FUNCTION "Analog I/O convert" : VOID
TITLE =ANALOGUE I/O MANAGEMENT
AUTHOR : Diego_M
VERSION : 0.1

BEGIN
NETWORK
TITLE =UR 0 Slot 5 Channel 0
//ENCODER PASS-LINE
      L     PED  272;
      DTR   ; // CONVERSION TO REAL
      T     LD    28;

      L     LD    28;
      L     2.856068e+007; // =0 mm IN ENCODER POINTS
      -R    ; // REAL mm IN ENCODER POINTS
      L     1.830000e-004; // =1 ENCODER POINT IN mm
      *R    ; // REAL mm PASS LINE
      T     "Data Block 12".MEASURE_PASS_LINE; // VISUALIZATION OP37
NETWORK
TITLE =UR 0 Slot 5 Channel 1
//                           ENCODER DIAMETER COIL
//THE COSTANT FOR CONVERSION IS THE RESULT OF THE MAXIMUM DIAMETER (1110mm) + THE
//MEASURE CALCULATED BY ENCODER POINTS AT UPPER LIMIT SWITCH (542,892619mm)
//THE POINT ENCODER (0,253333mm) IS NEGATIVE FOR DECREASING THE DIAMETER AS
//THE ENCODER INCREASES
      L     PED  276;
      DTR   ; // CONVERSION TO REAL
      T     LD    16;

      L     LD    16;
      L     -2.533330e-001; // 1 POINT ENCODER = mm
      *R    ; // DIAMETER MEASURE IN ENCODER POINTS
      L     1.653893e+003; // CONSTANT FOR CONVERSION IN REAL MEASURE
      +R    ; // REAL DIAMETER MEASURE
      T     "Data Block 12".COIL_DIAMETER_MEASURE; // MEASURE TO TD17
NETWORK
TITLE =UR 0 Slot 6 Channel 0
//CURRENT DECOILING

// Analog input reading
      CALL "SCALE" (
           IN                       := "400U1-A",
           HI_LIM                   := "Data Block 12".Hi_Lim_PEW288,
           LO_LIM                   := "Data Block 12".Lo_Lim_PEW288,
           BIPOLAR                  := TRUE,
           RET_VAL                  := "Data Block 12".Ret_Val_PEW288,
           OUT                      := "Data Block 12".Out_PEW288);



NETWORK
TITLE =UR 0 Slot 6 Channel 1
//ROUND PER MINUTE DECOILING
// Analog input reading
      CALL "SCALE" (
           IN                       := "400U1-V",
           HI_LIM                   := "Data Block 12".Hi_Lim_PEW290,
           LO_LIM                   := "Data Block 12".Lo_Lim_PEW290,
           BIPOLAR                  := TRUE,
           RET_VAL                  := "Data Block 12".Ret_Val_PEW290,
           OUT                      := "Data Block 12".Out_PEW290);


NETWORK
TITLE =UR 0 Slot 6 Channel 2
//ROUND PER MINUTE STRAIGHTENER
// Analog input reading
      CALL "SCALE" (
           IN                       := "411U1-A",
           HI_LIM                   := "Data Block 12".Hi_Lim_PEW292,
           LO_LIM                   := "Data Block 12".Lo_Lim_PEW292,
           BIPOLAR                  := TRUE,
           RET_VAL                  := "Data Block 12".Ret_Val_PEW292,
           OUT                      := "Data Block 12".Out_PEW292);



NETWORK
TITLE =UR 0 Slot 6 Channel 3
//CURRENT STRAIGHTENER
// Analog input reading
      CALL "SCALE" (
           IN                       := "411U1-V",
           HI_LIM                   := "Data Block 12".Hi_Lim_PEW294,
           LO_LIM                   := "Data Block 12".Lo_Lim_PEW294,
           BIPOLAR                  := TRUE,
           RET_VAL                  := "Data Block 12".Ret_Val_PEW294,
           OUT                      := "Data Block 12".Out_PEW294);


NETWORK
TITLE =UR 0 Slot 6 Channel 4
//COMPENETRATION ENTRY
      L     "423BQ1"; // 16 BIT ANALOGUE POINTS
      T     LD     0; // 32 BIT ANALOGUE POINTS
      DTR   ; // CONVERSION IN REAL
      T     LD     4; // REAL ANALOGUE POINTS
      L     2.554250e+004; // =0 ANALOGUE QUOTE
      -R    ; // REAL mm IN ANALOGUE POINTS
      L     5.400000e-003; // VALUE IN mm OF AN ANALOGUE POINT
      *R    ; // REAL mm
      T     "Data Block 12".Out_PEW296; // TD17 VISUALIZATION

NETWORK
TITLE =UR 0 Slot 6 Channel 5
//COMPENETRATION EXIT
      L     "423BQ2"; // 16 BIT ANALOGUE POINTS
      T     LD     8; // 32 BIT ANALOGUE POINTS
      DTR   ; // CONVERSION IN REAL
      T     LD    12; // REAL ANALOGUE POINTS
      L     2.554250e+004; // =0 ANALOGUE QUOTE
      -R    ; // REAL mm IN ANALOGUE POINTS
      L     5.400000e-003; // VALUE IN mm OF AN ANALOGUE POINT
      *R    ; // REAL mm
      T     "Data Block 12".Out_PEW298; // TD17 VISUALIZATION

NETWORK
TITLE =UR 0 Slot 6 Channel 6
//SPARE
// Analog input reading
      CALL "SCALE" (
           IN                       := PEW  300,
           HI_LIM                   := "Data Block 12".Hi_Lim_PEW300,
           LO_LIM                   := "Data Block 12".Lo_Lim_PEW300,
           BIPOLAR                  := FALSE,
           RET_VAL                  := "Data Block 12".Ret_Val_PEW300,
           OUT                      := "Data Block 12".Out_PEW300);

NETWORK
TITLE =UR 0 Slot 6 Channel 7
//SPARE
// Analog input reading
      CALL "SCALE" (
           IN                       := PEW  302,
           HI_LIM                   := "Data Block 12".Hi_Lim_PEW302,
           LO_LIM                   := "Data Block 12".Lo_Lim_PEW302,
           BIPOLAR                  := FALSE,
           RET_VAL                  := "Data Block 12".Ret_Val_PEW302,
           OUT                      := "Data Block 12".Out_PEW302);

NETWORK
TITLE =UR 0 Slot 7 Channel 0
//PROPORTIONAL VALVE FRONT MANDREL
// Analog output wraiting
      CALL "UNSCALE" (
           IN                       := "Data Block 12".In_PAW304,
           HI_LIM                   := "Data Block 12".Hi_Lim_PAW304,
           LO_LIM                   := "Data Block 12".Lo_Lim_PAW304,
           BIPOLAR                  := FALSE,
           RET_VAL                  := "Data Block 12".Ret_Val_PAW304,
           OUT                      := "386YV1");

NETWORK
TITLE =UR 0 Slot 7 Channel 1
//PROPORTIONAL VALVE REAR MANDREL
// Analog output wraiting
      CALL "UNSCALE" (
           IN                       := "Data Block 12".In_PAW306,
           HI_LIM                   := "Data Block 12".Hi_Lim_PAW306,
           LO_LIM                   := "Data Block 12".Lo_Lim_PAW306,
           BIPOLAR                  := FALSE,
           RET_VAL                  := "Data Block 12".Ret_Val_PAW306,
           OUT                      := "396YV1");

NETWORK
TITLE =UR 0 Slot 7 Channel 2
//TENSION DECOLING
// Analog output wraiting
      CALL "UNSCALE" (
           IN                       := "DATI ENCODER".Tiro,
           HI_LIM                   := "Data Block 12".Hi_Lim_PAW308,
           LO_LIM                   := "Data Block 12".Lo_Lim_PAW308,
           BIPOLAR                  := FALSE,
           RET_VAL                  := "Data Block 12".Ret_Val_PAW308,
           OUT                      := "AW308");

NETWORK
TITLE =UR 0 Slot 7 Channel 3
//SPEED STRAIGHTENER
// Analog output wraiting
      CALL "UNSCALE" (
           IN                       := "Data Block 12".In_PAW310,
           HI_LIM                   := "Data Block 12".Hi_Lim_PAW310,
           LO_LIM                   := "Data Block 12".Lo_Lim_PAW310,
           BIPOLAR                  := FALSE,
           RET_VAL                  := "Data Block 12".Ret_Val_PAW310,
           OUT                      := "AW310");

NETWORK
TITLE =UR 1 Slot 9 Channel 0
//SPEED FEEDER
// Analog output writing
      CALL "UNSCALE" (
           IN                       := "Data Block 12".In_PAW464,
           HI_LIM                   := "Data Block 12".Hi_Lim_PAW464,
           LO_LIM                   := "Data Block 12".Lo_Lim_PAW464,
           BIPOLAR                  := TRUE,
           RET_VAL                  := "Data Block 12".Ret_Val_PAW464,
           OUT                      := "AW464");

NETWORK
TITLE =UR 1 Slot 9 Channel 1
//DIAMETER COIL TO DECOILING
// Analog output wraiting
      L     PED  276;
      DTR   ; // CONVERSION TO REAL
      T     "Data Block 12".In_PAW466;

      U(    ;
      L     "Data Block 12".In_PAW466;
      L     3.000000e+003; // LOW LIMIT
      <R    ; // IF LOWER OF LIMIT
      )     ;
      SPBN  OFFS;
      L     3.000000e+003;
      T     "Data Block 12".In_PAW466;
OFFS: NOP   0;

      CALL "UNSCALE" (
           IN                       := "Data Block 12".In_PAW466,
           HI_LIM                   := "Data Block 12".Hi_Lim_PAW466,
           LO_LIM                   := "Data Block 12".Lo_Lim_PAW466,
           BIPOLAR                  := FALSE,
           RET_VAL                  := "Data Block 12".Ret_Val_PAW466,
           OUT                      := "Data Block 12".Out_PAW466);

      L     "Data Block 12".Out_PAW466;
      T     "AW466";


NETWORK
TITLE =UR 1 Slot 9 Channel 2
//WIDTH COIL TO DECOILING
// Analog output wraiting

      CALL "UNSCALE" (
           IN                       := "DATI ENCODER".LARG_COIL,
           HI_LIM                   := "Data Block 12".Hi_Lim_PAW468,
           LO_LIM                   := "Data Block 12".Lo_Lim_PAW468,
           BIPOLAR                  := FALSE,
           RET_VAL                  := "Data Block 12".Ret_Val_PAW468,
           OUT                      := "AW468");

NETWORK
TITLE =UR 1 Slot 9 Channel 3
//SPARE

// Analog output wraiting
      CALL "UNSCALE" (
           IN                       := "Data Block 12".In_PAW470,
           HI_LIM                   := "Data Block 12".Hi_Lim_PAW470,
           LO_LIM                   := "Data Block 12".Lo_Lim_PAW470,
           BIPOLAR                  := FALSE,
           RET_VAL                  := "Data Block 12".Ret_Val_PAW470,
           OUT                      := PAW  470);

NETWORK
TITLE =


      L     PED  272;
      T     "DATI ENCODER".STAT0; // pass line
//;
      L     PED  276;
      T     "DATI ENCODER".STAT1; // Diametro coils
//;
      L     "Data Block 12".Out_PEW294;
      T     "DATI ENCODER".STAT67; // Corrente motore spianatrice


END_FUNCTION

